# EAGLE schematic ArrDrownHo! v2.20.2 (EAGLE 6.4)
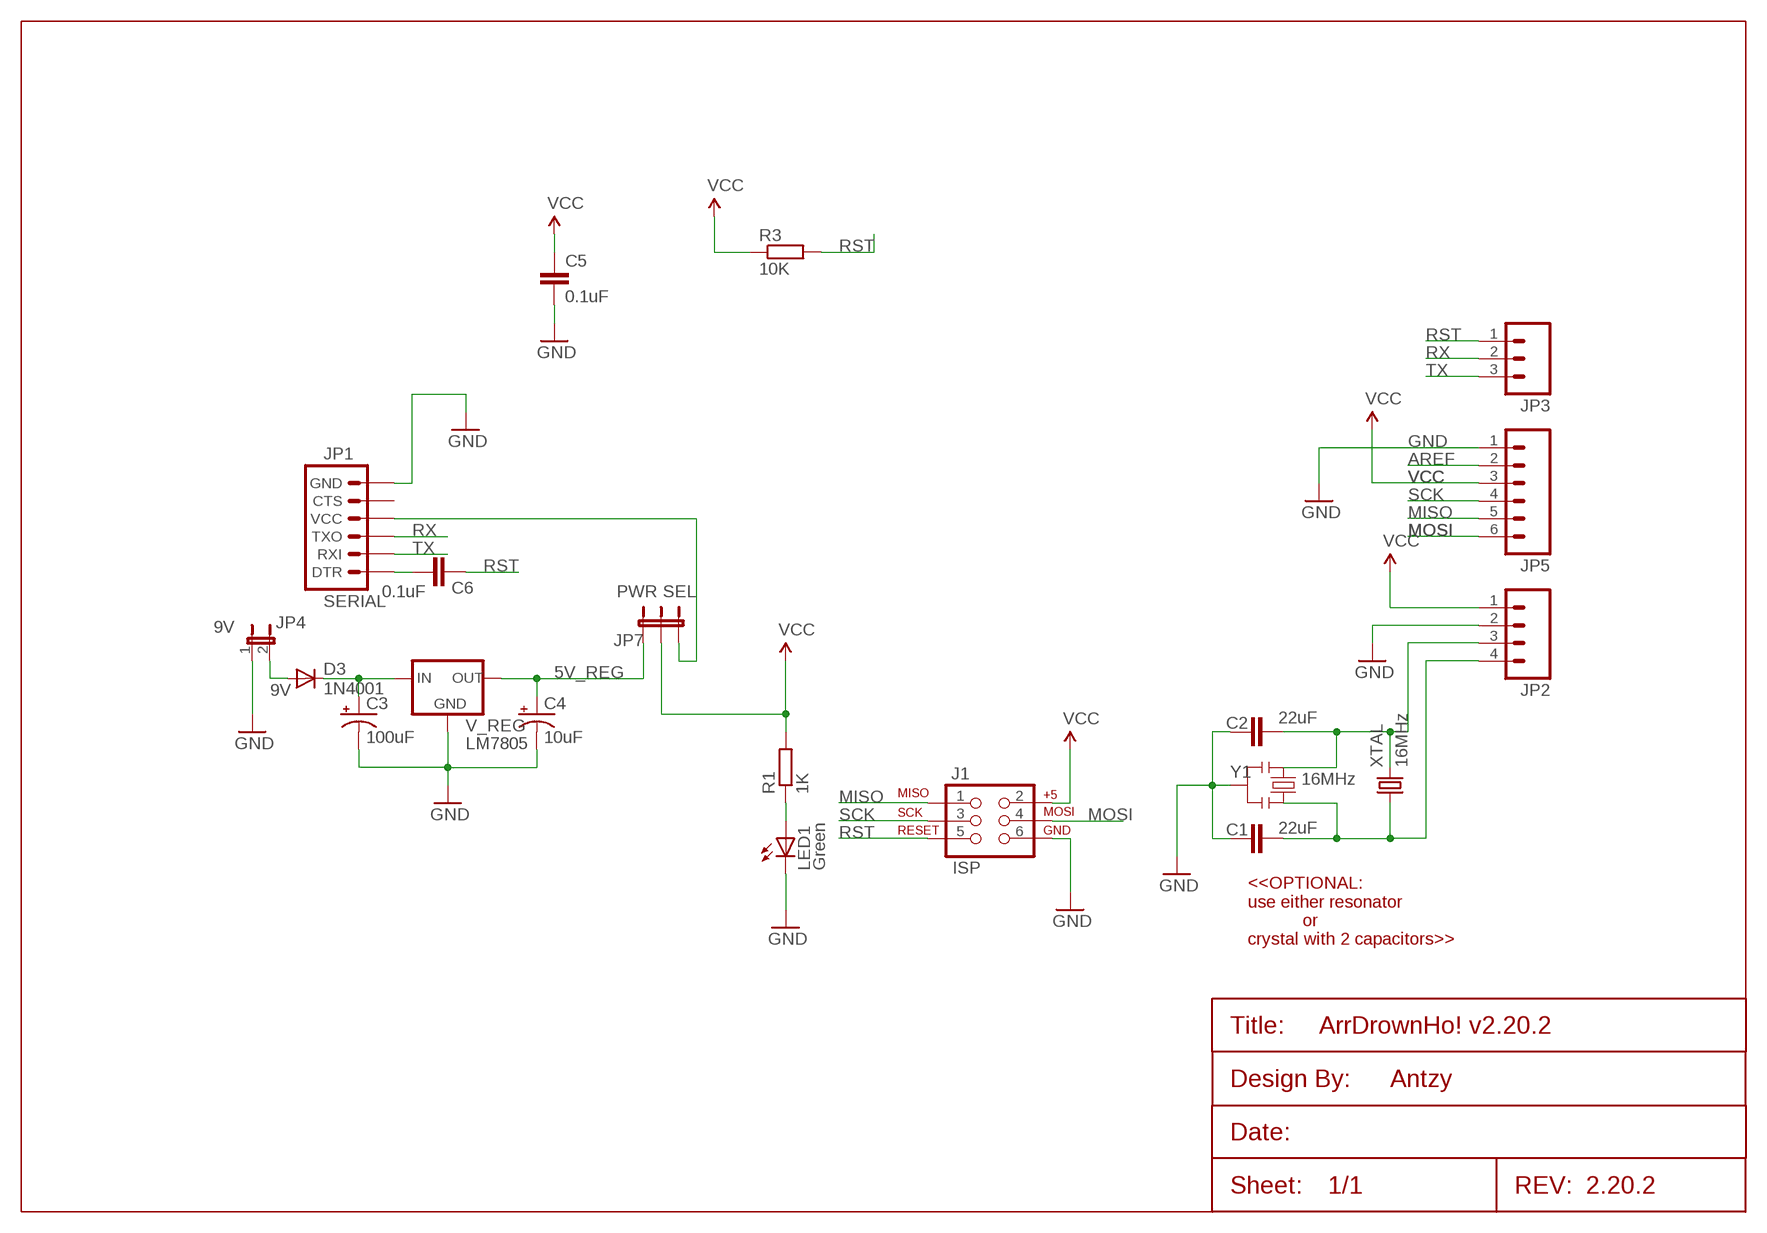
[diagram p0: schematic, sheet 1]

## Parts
C1  22uF  CAPEZ  [CAP-PTH-SMALLEZ]
C2  22uF  CAPEZ  [CAP-PTH-SMALLEZ]
C3  100uF  CAP_POLPTH1  [CPOL-RADIAL-100UF-25V]
C4  10uF  CAP_POLPTH2  [CPOL-RADIAL-10UF-25V]
C5  0.1uF  CAPPTH  [CAP-PTH-SMALL]
C6  0.1uF  CAPPTH  [CAP-PTH-SMALL]
D3  1N4001  DIODE-D-2.5  [D-2.5]
J1  ISP  AVR_SPI_PRG_6PTH  [2X3]
JP1  SERIAL  ARDUINO_SERIAL_PROGRAMPTH  [1X06]
JP2  M04PTH  [1X04]
JP3  M03PTH  [1X03]
JP4  9V  JUMPER-2PTH  [1X02]
JP5  M06SIP  [1X06]
JP7  PWR SEL  JUMPER-3PTH  [1X03]
LED1  Green  LED3MM  [LED3MM]
R1  1K  R-EU_0204/2V  [0204V]
R3  10K  R-EU_0204/2V  [0204V]
U$1  ANTZY_FRAME  [ANTZY_FRAME]
V_REG  LM7805  78XXS  [78XXS]
XTAL  16MHz  CRYSTALHC49US  [HC49US]
Y1  16MHz  RESONATORPTH  [RESONATOR-PTH]

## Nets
5V_REG: C4.1(+) JP7.1 V_REG.OUT
9V: D3.A JP4.2
AREF: JP5.2
GND: C1.1 C2.1 C3.2(-) C4.2(-) C5.2 J1.6 JP1.6(GND) JP2.2 JP4.1 JP5.1 LED1.K(C) V_REG.GND Y1.2
MISO: J1.1 JP5.5
MOSI: J1.4 JP5.6
N$1: C1.2 JP2.4 XTAL.1 Y1.3
N$2: C2.2 JP2.3 XTAL.2 Y1.1
N$3: JP1.4(VCC) JP7.3
N$4: C6.2 JP1.1(DTR)
N$5: LED1.A R1.1
N$13: C3.1(+) D3.C V_REG.IN
RST: C6.1 J1.5 JP3.1 R3.2
RX: JP1.3(TXO) JP3.2
SCK: J1.3 JP5.4
TX: JP1.2(RXI) JP3.3
VCC: C5.1 J1.2 JP2.1 JP5.3 JP7.2 R1.2 R3.1
Unconnected: JP1.5(CTS)

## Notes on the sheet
- <<OPTIONAL:
  use either resonator
             or
  crystal with 2 capacitors>>
- Antzy
- 2.20.2

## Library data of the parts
C1 C2 = SparkFun-Capacitors:CAP: Capacitor
C3 C4 = SparkFun-Passives:CAP_POL: Capacitor Polarized
C5 C6 = SparkFun-Passives:CAP: Capacitor
D3 = diode:DIODE-: DIODE
J1 = SparkFun-Connectors:AVR_SPI_PRG_6: AVR ISP 6 Pin This is the reduced ISP connector for AVR programming. Common on Arduino. This footprint will take up less PCB space and can be used with a 10-pin to 6-pin adapter such as SKU: BOB-08508
JP1 = SparkFun-Connectors:ARDUINO_SERIAL_PROGRAM: FTDI connector footprints
JP2 = SparkFun-Connectors:M04: Header 4 Standard 4-pin 0.1" header. Use with straight break away headers (SKU : PRT-00116), right angle break away headers (PRT-00553), swiss pins (PRT-00743), machine pins (PRT-00117), and female headers (PRT-00115). Molex polarized connector foot print use with SKU : PRT-08231 with associated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
JP3 = SparkFun-Connectors:M03: Header 3 Standard 3-pin 0.1" header. Use with straight break away headers (SKU : PRT-00116), right angle break away headers (PRT-00553), swiss pins (PRT-00743), machine pins (PRT-00117), and female headers (PRT-00115). Molex polarized connector foot print use with SKU : PRT-08232 with associated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
JP4 = SparkFun-Passives:JUMPER-2: Jumper
JP5 = SparkFun-Connectors:M06: Header 6 Standard 6-pin 0.1" header. Use with straight break away headers (SKU : PRT-00116), right angle break away headers (PRT-00553), swiss pins (PRT-00743), machine pins (PRT-00117), and female headers (PRT-00115). Molex polarized connector foot print use with SKU : PRT-08094 with associated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
JP7 = SparkFun-Passives:JUMPER-3
LED1 = SparkFun-LED:LED: LEDs
R1 R3 = resistor:R-EU_: RESISTOR, European symbol
U$1 = Antzy's stuff:ANTZY_FRAME
V_REG = v-reg:78XXS: VOLTAGE REGULATOR
XTAL = SparkFun-FreqCtrl:CRYSTAL: Various standard crystals. Proven footprints. Spark Fun Electronics SKU : COM-00534
Y1 = SparkFun-FreqCtrl:RESONATOR: Resonator Small SMD resonator. Used, eg, on the Arduino Pro/ Pro Mini boards. 8MHz- XTAL-08895 16MHz- XTAL-08900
